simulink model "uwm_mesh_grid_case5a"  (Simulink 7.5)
settings: Solver=ode45  StartTime=0.0  StopTime=3.0  RelTol=1e-4
undefined symbols (not defined in the file or in its folder): D1, Delta, dfilt, DiscIntNeverNeededParam, Discrete, no, powergui, steady, ZData
libraries: powerlib x259, powerlib_extras x68, dsparch4 x11
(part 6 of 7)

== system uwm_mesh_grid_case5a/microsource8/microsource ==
  Vpk : Inport  OutDataType=fixdt(1, 16)  OutScaling=2^0
  w : Inport  Port=2  OutDataType=fixdt(1, 16)  OutScaling=2^0
  Demux : Demux  Outputs=3
  Ground2 : powerlib/Elements/Ground  DialogController=POWERSYS.PowerSysDialog  PhysicalDomain=powersysdomain  SubClassName=unknown  LeftPortType=p1  RightPortType=p1  LConnTagsString=a
  Integrator : Integrator
  Mux : Mux  Inputs=3
  Product : Product  OutDataType=sfix(16)  OutScaling=2^0
  Series RLC Branch : powerlib/Elements/Series RLC Branch  DialogController=POWERSYS.PowerSysDialog  PhysicalDomain=powersysdomain  SubClassName=unknown  LeftPortType=p1  RightPortType=p1  LConnTagsString=__new0  RConnTagsString=__new0  BranchType=C  Resistance=1  Inductance=1e-3  SetiL0=off  InitialCurrent=0  Capacitance=1e-8  Setx0=off  InitialVoltage=0  Measurements=None
  phaseA : powerlib/Electrical Sources/Controlled Voltage Source  DialogController=POWERSYS.PowerSysDialog  SystemSampleTime=-1  Initialize=on  Source_Type=AC  Amplitude=0  Phase=0  Frequency=0  Measurements=None
  phaseB : powerlib/Electrical Sources/Controlled Voltage Source  DialogController=POWERSYS.PowerSysDialog  SystemSampleTime=-1  Initialize=on  Source_Type=AC  Amplitude=0  Phase=0  Frequency=0  Measurements=None
  phaseC : powerlib/Electrical Sources/Controlled Voltage Source  DialogController=POWERSYS.PowerSysDialog  SystemSampleTime=-1  Initialize=on  Source_Type=AC  Amplitude=0  Phase=0  Frequency=0  Measurements=None
  v_A : Fcn  Expr=cos(u)
  v_B : Fcn  Expr=cos(u-2*pi/3)
  v_C : Fcn  Expr=cos(u+2*pi/3)
  Va : PMIOPort  Tag=PMCPort  Port=1  Side=Right
  Vb : PMIOPort  Tag=PMCPort  Port=2  Side=Right
  Vc : PMIOPort  Tag=PMCPort  Port=3  Side=Right
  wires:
  Product/1 -> Demux/1
  Vpk/1 -> Product/1
  Mux/1 -> Product/2
  w/1 -> Integrator/1
  Integrator/1 -> v_A/1, v_B/1, v_C/1
  v_A/1 -> Mux/1
  v_B/1 -> Mux/2
  v_C/1 -> Mux/3
  Demux/1 -> phaseA/1
  Demux/2 -> phaseB/1
  Demux/3 -> phaseC/1
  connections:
  Vb/RConn1 -- phaseB/RConn1 -- phaseA/LConn1
  Va/RConn1 -- phaseC/LConn1 -- phaseA/RConn1
  Vc/RConn1 -- phaseC/RConn1
  Series RLC Branch/RConn1 -- Ground2/LConn1
  Series RLC Branch/LConn1 -- phaseB/LConn1

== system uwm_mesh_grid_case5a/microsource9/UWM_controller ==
  note: P
  note: Q
  v_meas : Inport
  i_meas : Inport  Port=2
  E_req : Inport  Port=3
  P_req : Inport  Port=4
  " pu convert P" : Gain  Gain=1/Sbase  ParameterDataType=sfix(16)  ParameterScaling=2^0  OutDataType=sfix(16)  OutScaling=2^0
  " pu convert S" : Gain  Gain=1/Sbase  ParameterDataType=sfix(16)  ParameterScaling=2^0  OutDataType=sfix(16)  OutScaling=2^0
  " pu convert V" : Gain  Gain=1/(Vbase/sqrt(3))  ParameterDataType=sfix(16)  ParameterScaling=2^0  OutDataType=sfix(16)  OutScaling=2^0
  3-phase  Instantaneous  Active & Reactive Power : powerlib_extras/Measurements/3-phase  Instantaneous  Active & Reactive Power  DialogController=POWERSYS.PowerSysDialog  SystemSampleTime=-1
  Demux : Demux  Outputs=2
  PI-Control : Subsystem
  RMS : Fcn  Expr=sqrt(u(1)*u(1)+u(2)*u(2)+u(3)*u(3))/sqrt(3)
  Sum : Sum  Inputs=|-+  OutDataType=sfix(16)  OutScaling=2^0
  Sum1 : Sum  Inputs=|+-  OutDataType=sfix(16)  OutScaling=2^0
  Sum2 : Sum  Inputs=+-|  OutDataType=sfix(16)  OutScaling=2^0
  Sum3 : Sum  Inputs=+++  OutDataType=sfix(16)  OutScaling=2^0
  Transfer Fcn : TransferFcn  Denominator=[.01 1]
  Transfer Fcn1 : TransferFcn  Denominator=[.01 1]
  Transfer Fcn2 : TransferFcn  Denominator=[.01 1]
  k : Gain  Gain=1/pi  ParameterDataType=sfix(16)  ParameterScaling=2^0  OutDataType=sfix(16)  OutScaling=2^0
  limiter : Subsystem
  mP droop : Gain  Gain=pi  ParameterDataType=sfix(16)  ParameterScaling=2^0  OutDataType=sfix(16)  OutScaling=2^0
  "mQ droop " : Gain  Gain=0.05  ParameterDataType=sfix(16)  ParameterScaling=2^0  OutDataType=sfix(16)  OutScaling=2^0
  w0 : Constant  Value=60*2*pi  OutDataType=fixdt(1, 16)  OutScaling=2^0
  Vpk : Outport
  w : Outport  Port=2
  Pmm : Outport  Port=3
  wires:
  Transfer Fcn2/1 -> " pu convert V"/1
  Transfer Fcn/1 -> " pu convert P"/1
  " pu convert P"/1 -> "mQ droop "/1
  Transfer Fcn1/1 -> " pu convert S"/1
  " pu convert S"/1 -> limiter/1(In1), Sum2/2
  i_meas/1 -> 3-phase  Instantaneous  Active & Reactive Power/2
  P_req/1 -> Sum2/1
  mP droop/1 -> Sum3/2
  limiter/1(Out1) -> Sum3/1, k/1
  w0/1 -> Sum3/3
  Sum2/1 -> mP droop/1
  Sum1/1 -> PI-Control/1(In1)
  Sum/1 -> Sum1/1
  "mQ droop "/1 -> Sum/1
  RMS/1 -> Transfer Fcn2/1
  Demux/2 -> Transfer Fcn/1
  Demux/1 -> Transfer Fcn1/1
  3-phase  Instantaneous  Active & Reactive Power/1 -> Demux/1
  v_meas/1 -> RMS/1, 3-phase  Instantaneous  Active & Reactive Power/1
  PI-Control/1(Out1) -> Vpk/1
  Sum3/1 -> w/1
  E_req/1 -> Sum/2
  " pu convert V"/1 -> Sum1/2
  k/1 -> Pmm/1

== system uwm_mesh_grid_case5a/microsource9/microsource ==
  Vpk : Inport  OutDataType=fixdt(1, 16)  OutScaling=2^0
  w : Inport  Port=2  OutDataType=fixdt(1, 16)  OutScaling=2^0
  Demux : Demux  Outputs=3
  Ground2 : powerlib/Elements/Ground  DialogController=POWERSYS.PowerSysDialog  PhysicalDomain=powersysdomain  SubClassName=unknown  LeftPortType=p1  RightPortType=p1  LConnTagsString=a
  Integrator : Integrator
  Mux : Mux  Inputs=3
  Product : Product  OutDataType=sfix(16)  OutScaling=2^0
  Series RLC Branch : powerlib/Elements/Series RLC Branch  DialogController=POWERSYS.PowerSysDialog  PhysicalDomain=powersysdomain  SubClassName=unknown  LeftPortType=p1  RightPortType=p1  LConnTagsString=__new0  RConnTagsString=__new0  BranchType=C  Resistance=1  Inductance=1e-3  SetiL0=off  InitialCurrent=0  Capacitance=1e-8  Setx0=off  InitialVoltage=0  Measurements=None
  phaseA : powerlib/Electrical Sources/Controlled Voltage Source  DialogController=POWERSYS.PowerSysDialog  SystemSampleTime=-1  Initialize=on  Source_Type=AC  Amplitude=0  Phase=0  Frequency=0  Measurements=None
  phaseB : powerlib/Electrical Sources/Controlled Voltage Source  DialogController=POWERSYS.PowerSysDialog  SystemSampleTime=-1  Initialize=on  Source_Type=AC  Amplitude=0  Phase=0  Frequency=0  Measurements=None
  phaseC : powerlib/Electrical Sources/Controlled Voltage Source  DialogController=POWERSYS.PowerSysDialog  SystemSampleTime=-1  Initialize=on  Source_Type=AC  Amplitude=0  Phase=0  Frequency=0  Measurements=None
  v_A : Fcn  Expr=cos(u)
  v_B : Fcn  Expr=cos(u-2*pi/3)
  v_C : Fcn  Expr=cos(u+2*pi/3)
  Va : PMIOPort  Tag=PMCPort  Port=1  Side=Right
  Vb : PMIOPort  Tag=PMCPort  Port=2  Side=Right
  Vc : PMIOPort  Tag=PMCPort  Port=3  Side=Right
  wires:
  Product/1 -> Demux/1
  Vpk/1 -> Product/1
  Mux/1 -> Product/2
  w/1 -> Integrator/1
  Integrator/1 -> v_A/1, v_B/1, v_C/1
  v_A/1 -> Mux/1
  v_B/1 -> Mux/2
  v_C/1 -> Mux/3
  Demux/1 -> phaseA/1
  Demux/2 -> phaseB/1
  Demux/3 -> phaseC/1
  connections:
  Vb/RConn1 -- phaseB/RConn1 -- phaseA/LConn1
  Va/RConn1 -- phaseC/LConn1 -- phaseA/RConn1
  Vc/RConn1 -- phaseC/RConn1
  Series RLC Branch/RConn1 -- Ground2/LConn1
  Series RLC Branch/LConn1 -- phaseB/LConn1

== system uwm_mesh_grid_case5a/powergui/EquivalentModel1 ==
  Gates : Subsystem
  Sources : Subsystem
  State-Space : S-Function  FunctionName=sfun_spssw_discc  Parameters=S.Ts,S.A, S.B, S.C, S.D, S.x0, S.EnableUseOfTLC,S.SwitchResistance ,S.SwitchType, S.SwitchGateInitialValue, S.OutputsToResetToZero  EnableBusSupport=off
  Status : Subsystem
  Yout : Subsystem
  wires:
  State-Space/1 -> Yout/1(v,i)
  State-Space/2 -> Status/1(status)
  Sources/1(u) -> State-Space/1
  Gates/1(gates) -> State-Space/2

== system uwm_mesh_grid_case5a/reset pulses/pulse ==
  Step : Step  Time=tstart  SampleTime=0
  Step1 : Step  Time=tstart+dt  After=-1  SampleTime=0
  Sum : Sum  Inputs=|++  OutDataType=fixdt(1, 16)  OutScaling=2^0
  Out1 : Outport
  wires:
  Step/1 -> Sum/2
  Step1/1 -> Sum/1
  Sum/1 -> Out1/1

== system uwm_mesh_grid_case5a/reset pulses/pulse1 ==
  Step : Step  Time=tstart  SampleTime=0
  Step1 : Step  Time=tstart+dt  After=-1  SampleTime=0
  Sum : Sum  Inputs=|++  OutDataType=fixdt(1, 16)  OutScaling=2^0
  Out1 : Outport
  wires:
  Step/1 -> Sum/2
  Step1/1 -> Sum/1
  Sum/1 -> Out1/1

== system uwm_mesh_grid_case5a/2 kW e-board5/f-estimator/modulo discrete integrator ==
  In1 : Inport
  Abs : Abs
  Constant1 : Constant  OutDataType=sfix(16)  OutScaling=2^0
  Discrete-Time Integrator : DiscreteIntegrator  ExternalReset=rising  InitialConditionSource=external  SampleTime=dt  OutDataType=fixdt(1, 16)  OutScaling=2^0  UpperSaturationLimit=100  LowerSaturationLimit=-100  ShowStatePort=on  ICPrevOutput=DiscIntNeverNeededParam  ICPrevScaledInput=DiscIntNeverNeededParam
  Gain1 : Gain  Gain=1+.0001  ParameterDataType=sfix(16)  ParameterScaling=2^0  OutDataType=sfix(16)  OutScaling=2^0
  IC : InitialCondition  Value=0
  Math Function : Math  Operator=rem  OutDataType=sfix(16)  OutScaling=2^0
  Relational Operator : RelationalOperator
  Out1 : Outport
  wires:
  Math Function/1 -> IC/1
  IC/1 -> Discrete-Time Integrator/3
  Discrete-Time Integrator/1 -> Out1/1
  In1/1 -> Discrete-Time Integrator/1
  Abs/1 -> Math Function/1, Relational Operator/1
  Constant1/1 -> Math Function/2, Relational Operator/2
  Gain1/1 -> Abs/1
  Discrete-Time Integrator/State -> Gain1/1
  Relational Operator/1 -> Discrete-Time Integrator/2

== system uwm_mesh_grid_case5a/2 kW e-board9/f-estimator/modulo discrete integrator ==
  In1 : Inport
  Abs : Abs
  Constant1 : Constant  OutDataType=sfix(16)  OutScaling=2^0
  Discrete-Time Integrator : DiscreteIntegrator  ExternalReset=rising  InitialConditionSource=external  SampleTime=dt  OutDataType=fixdt(1, 16)  OutScaling=2^0  UpperSaturationLimit=100  LowerSaturationLimit=-100  ShowStatePort=on  ICPrevOutput=DiscIntNeverNeededParam  ICPrevScaledInput=DiscIntNeverNeededParam
  Gain1 : Gain  Gain=1+.0001  ParameterDataType=sfix(16)  ParameterScaling=2^0  OutDataType=sfix(16)  OutScaling=2^0
  IC : InitialCondition  Value=0
  Math Function : Math  Operator=rem  OutDataType=sfix(16)  OutScaling=2^0
  Relational Operator : RelationalOperator
  Out1 : Outport
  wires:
  Math Function/1 -> IC/1
  IC/1 -> Discrete-Time Integrator/3
  Discrete-Time Integrator/1 -> Out1/1
  In1/1 -> Discrete-Time Integrator/1
  Abs/1 -> Math Function/1, Relational Operator/1
  Constant1/1 -> Math Function/2, Relational Operator/2
  Gain1/1 -> Abs/1
  Discrete-Time Integrator/State -> Gain1/1
  Relational Operator/1 -> Discrete-Time Integrator/2

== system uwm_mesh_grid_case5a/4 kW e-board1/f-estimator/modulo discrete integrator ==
  In1 : Inport
  Abs : Abs
  Constant1 : Constant  OutDataType=sfix(16)  OutScaling=2^0
  Discrete-Time Integrator : DiscreteIntegrator  ExternalReset=rising  InitialConditionSource=external  SampleTime=dt  OutDataType=fixdt(1, 16)  OutScaling=2^0  UpperSaturationLimit=100  LowerSaturationLimit=-100  ShowStatePort=on  ICPrevOutput=DiscIntNeverNeededParam  ICPrevScaledInput=DiscIntNeverNeededParam
  Gain1 : Gain  Gain=1+.0001  ParameterDataType=sfix(16)  ParameterScaling=2^0  OutDataType=sfix(16)  OutScaling=2^0
  IC : InitialCondition  Value=0
  Math Function : Math  Operator=rem  OutDataType=sfix(16)  OutScaling=2^0
  Relational Operator : RelationalOperator
  Out1 : Outport
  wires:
  Math Function/1 -> IC/1
  IC/1 -> Discrete-Time Integrator/3
  Discrete-Time Integrator/1 -> Out1/1
  In1/1 -> Discrete-Time Integrator/1
  Abs/1 -> Math Function/1, Relational Operator/1
  Constant1/1 -> Math Function/2, Relational Operator/2
  Gain1/1 -> Abs/1
  Discrete-Time Integrator/State -> Gain1/1
  Relational Operator/1 -> Discrete-Time Integrator/2

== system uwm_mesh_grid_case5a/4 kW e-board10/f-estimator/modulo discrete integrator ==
  In1 : Inport
  Abs : Abs
  Constant1 : Constant  OutDataType=sfix(16)  OutScaling=2^0
  Discrete-Time Integrator : DiscreteIntegrator  ExternalReset=rising  InitialConditionSource=external  SampleTime=dt  OutDataType=fixdt(1, 16)  OutScaling=2^0  UpperSaturationLimit=100  LowerSaturationLimit=-100  ShowStatePort=on  ICPrevOutput=DiscIntNeverNeededParam  ICPrevScaledInput=DiscIntNeverNeededParam
  Gain1 : Gain  Gain=1+.0001  ParameterDataType=sfix(16)  ParameterScaling=2^0  OutDataType=sfix(16)  OutScaling=2^0
  IC : InitialCondition  Value=0
  Math Function : Math  Operator=rem  OutDataType=sfix(16)  OutScaling=2^0
  Relational Operator : RelationalOperator
  Out1 : Outport
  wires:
  Math Function/1 -> IC/1
  IC/1 -> Discrete-Time Integrator/3
  Discrete-Time Integrator/1 -> Out1/1
  In1/1 -> Discrete-Time Integrator/1
  Abs/1 -> Math Function/1, Relational Operator/1
  Constant1/1 -> Math Function/2, Relational Operator/2
  Gain1/1 -> Abs/1
  Discrete-Time Integrator/State -> Gain1/1
  Relational Operator/1 -> Discrete-Time Integrator/2

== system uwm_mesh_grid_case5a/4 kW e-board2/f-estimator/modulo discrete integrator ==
  In1 : Inport
  Abs : Abs
  Constant1 : Constant  OutDataType=sfix(16)  OutScaling=2^0
  Discrete-Time Integrator : DiscreteIntegrator  ExternalReset=rising  InitialConditionSource=external  SampleTime=dt  OutDataType=fixdt(1, 16)  OutScaling=2^0  UpperSaturationLimit=100  LowerSaturationLimit=-100  ShowStatePort=on  ICPrevOutput=DiscIntNeverNeededParam  ICPrevScaledInput=DiscIntNeverNeededParam
  Gain1 : Gain  Gain=1+.0001  ParameterDataType=sfix(16)  ParameterScaling=2^0  OutDataType=sfix(16)  OutScaling=2^0
  IC : InitialCondition  Value=0
  Math Function : Math  Operator=rem  OutDataType=sfix(16)  OutScaling=2^0
  Relational Operator : RelationalOperator
  Out1 : Outport
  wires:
  Math Function/1 -> IC/1
  IC/1 -> Discrete-Time Integrator/3
  Discrete-Time Integrator/1 -> Out1/1
  In1/1 -> Discrete-Time Integrator/1
  Abs/1 -> Math Function/1, Relational Operator/1
  Constant1/1 -> Math Function/2, Relational Operator/2
  Gain1/1 -> Abs/1
  Discrete-Time Integrator/State -> Gain1/1
  Relational Operator/1 -> Discrete-Time Integrator/2

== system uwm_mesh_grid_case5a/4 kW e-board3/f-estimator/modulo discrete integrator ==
  In1 : Inport
  Abs : Abs
  Constant1 : Constant  OutDataType=sfix(16)  OutScaling=2^0
  Discrete-Time Integrator : DiscreteIntegrator  ExternalReset=rising  InitialConditionSource=external  SampleTime=dt  OutDataType=fixdt(1, 16)  OutScaling=2^0  UpperSaturationLimit=100  LowerSaturationLimit=-100  ShowStatePort=on  ICPrevOutput=DiscIntNeverNeededParam  ICPrevScaledInput=DiscIntNeverNeededParam
  Gain1 : Gain  Gain=1+.0001  ParameterDataType=sfix(16)  ParameterScaling=2^0  OutDataType=sfix(16)  OutScaling=2^0
  IC : InitialCondition  Value=0
  Math Function : Math  Operator=rem  OutDataType=sfix(16)  OutScaling=2^0
  Relational Operator : RelationalOperator
  Out1 : Outport
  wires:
  Math Function/1 -> IC/1
  IC/1 -> Discrete-Time Integrator/3
  Discrete-Time Integrator/1 -> Out1/1
  In1/1 -> Discrete-Time Integrator/1
  Abs/1 -> Math Function/1, Relational Operator/1
  Constant1/1 -> Math Function/2, Relational Operator/2
  Gain1/1 -> Abs/1
  Discrete-Time Integrator/State -> Gain1/1
  Relational Operator/1 -> Discrete-Time Integrator/2

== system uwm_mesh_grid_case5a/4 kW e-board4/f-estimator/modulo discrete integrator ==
  In1 : Inport
  Abs : Abs
  Constant1 : Constant  OutDataType=sfix(16)  OutScaling=2^0
  Discrete-Time Integrator : DiscreteIntegrator  ExternalReset=rising  InitialConditionSource=external  SampleTime=dt  OutDataType=fixdt(1, 16)  OutScaling=2^0  UpperSaturationLimit=100  LowerSaturationLimit=-100  ShowStatePort=on  ICPrevOutput=DiscIntNeverNeededParam  ICPrevScaledInput=DiscIntNeverNeededParam
  Gain1 : Gain  Gain=1+.0001  ParameterDataType=sfix(16)  ParameterScaling=2^0  OutDataType=sfix(16)  OutScaling=2^0
  IC : InitialCondition  Value=0
  Math Function : Math  Operator=rem  OutDataType=sfix(16)  OutScaling=2^0
  Relational Operator : RelationalOperator
  Out1 : Outport
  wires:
  Math Function/1 -> IC/1
  IC/1 -> Discrete-Time Integrator/3
  Discrete-Time Integrator/1 -> Out1/1
  In1/1 -> Discrete-Time Integrator/1
  Abs/1 -> Math Function/1, Relational Operator/1
  Constant1/1 -> Math Function/2, Relational Operator/2
  Gain1/1 -> Abs/1
  Discrete-Time Integrator/State -> Gain1/1
  Relational Operator/1 -> Discrete-Time Integrator/2

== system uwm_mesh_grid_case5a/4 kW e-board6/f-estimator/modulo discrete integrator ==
  In1 : Inport
  Abs : Abs
  Constant1 : Constant  OutDataType=sfix(16)  OutScaling=2^0
  Discrete-Time Integrator : DiscreteIntegrator  ExternalReset=rising  InitialConditionSource=external  SampleTime=dt  OutDataType=fixdt(1, 16)  OutScaling=2^0  UpperSaturationLimit=100  LowerSaturationLimit=-100  ShowStatePort=on  ICPrevOutput=DiscIntNeverNeededParam  ICPrevScaledInput=DiscIntNeverNeededParam
  Gain1 : Gain  Gain=1+.0001  ParameterDataType=sfix(16)  ParameterScaling=2^0  OutDataType=sfix(16)  OutScaling=2^0
  IC : InitialCondition  Value=0
  Math Function : Math  Operator=rem  OutDataType=sfix(16)  OutScaling=2^0
  Relational Operator : RelationalOperator
  Out1 : Outport
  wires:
  Math Function/1 -> IC/1
  IC/1 -> Discrete-Time Integrator/3
  Discrete-Time Integrator/1 -> Out1/1
  In1/1 -> Discrete-Time Integrator/1
  Abs/1 -> Math Function/1, Relational Operator/1
  Constant1/1 -> Math Function/2, Relational Operator/2
  Gain1/1 -> Abs/1
  Discrete-Time Integrator/State -> Gain1/1
  Relational Operator/1 -> Discrete-Time Integrator/2

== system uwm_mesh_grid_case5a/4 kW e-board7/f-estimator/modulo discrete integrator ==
  In1 : Inport
  Abs : Abs
  Constant1 : Constant  OutDataType=sfix(16)  OutScaling=2^0
  Discrete-Time Integrator : DiscreteIntegrator  ExternalReset=rising  InitialConditionSource=external  SampleTime=dt  OutDataType=fixdt(1, 16)  OutScaling=2^0  UpperSaturationLimit=100  LowerSaturationLimit=-100  ShowStatePort=on  ICPrevOutput=DiscIntNeverNeededParam  ICPrevScaledInput=DiscIntNeverNeededParam
  Gain1 : Gain  Gain=1+.0001  ParameterDataType=sfix(16)  ParameterScaling=2^0  OutDataType=sfix(16)  OutScaling=2^0
  IC : InitialCondition  Value=0
  Math Function : Math  Operator=rem  OutDataType=sfix(16)  OutScaling=2^0
  Relational Operator : RelationalOperator
  Out1 : Outport
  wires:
  Math Function/1 -> IC/1
  IC/1 -> Discrete-Time Integrator/3
  Discrete-Time Integrator/1 -> Out1/1
  In1/1 -> Discrete-Time Integrator/1
  Abs/1 -> Math Function/1, Relational Operator/1
  Constant1/1 -> Math Function/2, Relational Operator/2
  Gain1/1 -> Abs/1
  Discrete-Time Integrator/State -> Gain1/1
  Relational Operator/1 -> Discrete-Time Integrator/2

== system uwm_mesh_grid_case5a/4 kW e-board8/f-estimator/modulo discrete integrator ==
  In1 : Inport
  Abs : Abs
  Constant1 : Constant  OutDataType=sfix(16)  OutScaling=2^0
  Discrete-Time Integrator : DiscreteIntegrator  ExternalReset=rising  InitialConditionSource=external  SampleTime=dt  OutDataType=fixdt(1, 16)  OutScaling=2^0  UpperSaturationLimit=100  LowerSaturationLimit=-100  ShowStatePort=on  ICPrevOutput=DiscIntNeverNeededParam  ICPrevScaledInput=DiscIntNeverNeededParam
  Gain1 : Gain  Gain=1+.0001  ParameterDataType=sfix(16)  ParameterScaling=2^0  OutDataType=sfix(16)  OutScaling=2^0
  IC : InitialCondition  Value=0
  Math Function : Math  Operator=rem  OutDataType=sfix(16)  OutScaling=2^0
  Relational Operator : RelationalOperator
  Out1 : Outport
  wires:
  Math Function/1 -> IC/1
  IC/1 -> Discrete-Time Integrator/3
  Discrete-Time Integrator/1 -> Out1/1
  In1/1 -> Discrete-Time Integrator/1
  Abs/1 -> Math Function/1, Relational Operator/1
  Constant1/1 -> Math Function/2, Relational Operator/2
  Gain1/1 -> Abs/1
  Discrete-Time Integrator/State -> Gain1/1
  Relational Operator/1 -> Discrete-Time Integrator/2

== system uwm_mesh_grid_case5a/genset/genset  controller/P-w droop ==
  note: P
  P_req : Inport
  P : Inport  Port=2
  Sum2 : Sum  Inputs=+-|  OutDataType=sfix(16)  OutScaling=2^0
  Sum3 : Sum  Inputs=+++  OutDataType=sfix(16)  OutScaling=2^0
  k : Gain  Gain=1/pi  ParameterDataType=sfix(16)  ParameterScaling=2^0  OutDataType=sfix(16)  OutScaling=2^0
  limiter : Subsystem
  mP droop : Gain  Gain=pi  ParameterDataType=sfix(16)  ParameterScaling=2^0  OutDataType=sfix(16)  OutScaling=2^0
  rad2pu : Gain  Gain=1/(2*pi*60)  ParameterDataType=sfix(16)  ParameterScaling=2^0  OutDataType=sfix(16)  OutScaling=2^0
  w0 : Constant  Value=60*2*pi  OutDataType=fixdt(1, 16)  OutScaling=2^0
  w : Outport
  Pmm : Outport  Port=2
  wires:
  P_req/1 -> Sum2/1
  mP droop/1 -> Sum3/2
  limiter/1(Out1) -> Sum3/1, k/1
  w0/1 -> Sum3/3
  Sum2/1 -> mP droop/1
  P/1 -> limiter/1(In1), Sum2/2
  Sum3/1 -> rad2pu/1
  rad2pu/1 -> w/1
  k/1 -> Pmm/1

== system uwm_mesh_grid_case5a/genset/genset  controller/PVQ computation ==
  note: P
  note: Q
  Vabc : Inport  OutDataType=fixdt(1, 16)  OutScaling=2^0
  Iabc : Inport  Port=2  OutDataType=fixdt(1, 16)  OutScaling=2^0
  " pu convert P" : Gain  Gain=1/Sbase  ParameterDataType=sfix(16)  ParameterScaling=2^0  OutDataType=sfix(16)  OutScaling=2^0
  " pu convert S" : Gain  Gain=1/Sbase  ParameterDataType=sfix(16)  ParameterScaling=2^0  OutDataType=sfix(16)  OutScaling=2^0
  " pu convert V" : Gain  Gain=1/(Vbase/sqrt(3))  ParameterDataType=sfix(16)  ParameterScaling=2^0  OutDataType=sfix(16)  OutScaling=2^0
  3-phase  Instantaneous  Active & Reactive Power : powerlib_extras/Measurements/3-phase  Instantaneous  Active & Reactive Power  DialogController=POWERSYS.PowerSysDialog  SystemSampleTime=-1
  Demux : Demux  Outputs=2
  RMS : Fcn  Expr=sqrt(u(1)*u(1)+u(2)*u(2)+u(3)*u(3))/sqrt(3)
  Transfer Fcn1 : TransferFcn  Denominator=[.01 1]
  Transfer Fcn2 : TransferFcn  Denominator=[.01 1]
  Transfer Fcn3 : TransferFcn  Denominator=[.01 1]
  P_pu : Outport  OutDataType=fixdt(1, 16)  OutScaling=2^0
  Vt : Outport  Port=2  OutDataType=fixdt(1, 16)  OutScaling=2^0
  Q_pu : Outport  Port=3  OutDataType=fixdt(1, 16)  OutScaling=2^0
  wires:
  Iabc/1 -> 3-phase  Instantaneous  Active & Reactive Power/2
  RMS/1 -> " pu convert V"/1
  Demux/2 -> " pu convert P"/1
  Demux/1 -> " pu convert S"/1
  3-phase  Instantaneous  Active & Reactive Power/1 -> Demux/1
  Vabc/1 -> RMS/1, 3-phase  Instantaneous  Active & Reactive Power/1
  Transfer Fcn1/1 -> P_pu/1
  " pu convert S"/1 -> Transfer Fcn1/1
  Transfer Fcn2/1 -> Q_pu/1
  " pu convert P"/1 -> Transfer Fcn2/1
  Transfer Fcn3/1 -> Vt/1
  " pu convert V"/1 -> Transfer Fcn3/1

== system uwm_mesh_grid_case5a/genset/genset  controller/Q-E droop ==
  note: Q
  v_meas : Inport
  Q : Inport  Port=2
  E_req : Inport  Port=3
  PI-Control : Subsystem
  Sum : Sum  Inputs=|-+  OutDataType=sfix(16)  OutScaling=2^0
  Sum1 : Sum  Inputs=|+-  OutDataType=sfix(16)  OutScaling=2^0
  "mQ droop " : Gain  Gain=0.05  ParameterDataType=sfix(16)  ParameterScaling=2^0  OutDataType=sfix(16)  OutScaling=2^0
  Vpk : Outport
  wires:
  Sum1/1 -> PI-Control/1(In1)
  Sum/1 -> Sum1/1
  "mQ droop "/1 -> Sum/1
  PI-Control/1(Out1) -> Vpk/1
  Q/1 -> "mQ droop "/1
  E_req/1 -> Sum/2
  v_meas/1 -> Sum1/2

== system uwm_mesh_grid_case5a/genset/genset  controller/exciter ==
  wr : Inport  OutDataType=fixdt(1, 16)  OutScaling=2^0
  Ef_mcd_wr : Inport  Port=2  OutDataType=fixdt(1, 16)  OutScaling=2^0
  Product : Product  OutDataType=fixdt(1, 16)  OutScaling=2^0
  Saturation : Saturate  UpperLimit=10  LowerLimit=-10  OutDataType=fixdt(1, 16)  OutScaling=2^0
  Transfer Fcn : TransferFcn  Denominator=[.001 1]
  Ef : Outport  OutDataType=fixdt(1, 16)  OutScaling=2^0
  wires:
  wr/1 -> Product/2
  Ef_mcd_wr/1 -> Product/1
  Product/1 -> Saturation/1
  Saturation/1 -> Transfer Fcn/1
  Transfer Fcn/1 -> Ef/1

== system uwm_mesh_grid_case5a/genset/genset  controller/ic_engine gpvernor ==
  wr : Inport  OutDataType=fixdt(1, 16)  OutScaling=2^0
  Pmeas : Inport  Port=2  OutDataType=fixdt(1, 16)  OutScaling=2^0
  w : Inport  Port=3  OutDataType=fixdt(1, 16)  OutScaling=2^0
  IC_engine : Subsystem
  governor : Subsystem
  Pmech : Outport  OutDataType=fixdt(1, 16)  OutScaling=2^0
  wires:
  governor/1(fuel_cmd) -> IC_engine/1(fuel_cmd)
  Pmeas/1 -> governor/1(Pmeas)
  IC_engine/1(Pmech) -> Pmech/1
  wr/1 -> governor/3(wr), IC_engine/2(wr)
  w/1 -> governor/2(w)

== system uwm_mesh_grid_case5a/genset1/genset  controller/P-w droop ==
  note: P
  P_req : Inport
  P : Inport  Port=2
  Sum2 : Sum  Inputs=+-|  OutDataType=sfix(16)  OutScaling=2^0
  Sum3 : Sum  Inputs=+++  OutDataType=sfix(16)  OutScaling=2^0
  k : Gain  Gain=1/pi  ParameterDataType=sfix(16)  ParameterScaling=2^0  OutDataType=sfix(16)  OutScaling=2^0
  limiter : Subsystem
  mP droop : Gain  Gain=pi  ParameterDataType=sfix(16)  ParameterScaling=2^0  OutDataType=sfix(16)  OutScaling=2^0
  rad2pu : Gain  Gain=1/(2*pi*60)  ParameterDataType=sfix(16)  ParameterScaling=2^0  OutDataType=sfix(16)  OutScaling=2^0
  w0 : Constant  Value=60*2*pi  OutDataType=fixdt(1, 16)  OutScaling=2^0
  w : Outport
  Pmm : Outport  Port=2
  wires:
  P_req/1 -> Sum2/1
  mP droop/1 -> Sum3/2
  limiter/1(Out1) -> Sum3/1, k/1
  w0/1 -> Sum3/3
  Sum2/1 -> mP droop/1
  P/1 -> limiter/1(In1), Sum2/2
  Sum3/1 -> rad2pu/1
  rad2pu/1 -> w/1
  k/1 -> Pmm/1

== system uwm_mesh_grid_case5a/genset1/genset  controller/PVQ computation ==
  note: P
  note: Q
  Vabc : Inport  OutDataType=fixdt(1, 16)  OutScaling=2^0
  Iabc : Inport  Port=2  OutDataType=fixdt(1, 16)  OutScaling=2^0
  " pu convert P" : Gain  Gain=1/Sbase  ParameterDataType=sfix(16)  ParameterScaling=2^0  OutDataType=sfix(16)  OutScaling=2^0
  " pu convert S" : Gain  Gain=1/Sbase  ParameterDataType=sfix(16)  ParameterScaling=2^0  OutDataType=sfix(16)  OutScaling=2^0
  " pu convert V" : Gain  Gain=1/(Vbase/sqrt(3))  ParameterDataType=sfix(16)  ParameterScaling=2^0  OutDataType=sfix(16)  OutScaling=2^0
  3-phase  Instantaneous  Active & Reactive Power : powerlib_extras/Measurements/3-phase  Instantaneous  Active & Reactive Power  DialogController=POWERSYS.PowerSysDialog  SystemSampleTime=-1
  Demux : Demux  Outputs=2
  RMS : Fcn  Expr=sqrt(u(1)*u(1)+u(2)*u(2)+u(3)*u(3))/sqrt(3)
  Transfer Fcn1 : TransferFcn  Denominator=[.01 1]
  Transfer Fcn2 : TransferFcn  Denominator=[.01 1]
  Transfer Fcn3 : TransferFcn  Denominator=[.01 1]
  P_pu : Outport  OutDataType=fixdt(1, 16)  OutScaling=2^0
  Vt : Outport  Port=2  OutDataType=fixdt(1, 16)  OutScaling=2^0
  Q_pu : Outport  Port=3  OutDataType=fixdt(1, 16)  OutScaling=2^0
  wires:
  Iabc/1 -> 3-phase  Instantaneous  Active & Reactive Power/2
  RMS/1 -> " pu convert V"/1
  Demux/2 -> " pu convert P"/1
  Demux/1 -> " pu convert S"/1
  3-phase  Instantaneous  Active & Reactive Power/1 -> Demux/1
  Vabc/1 -> RMS/1, 3-phase  Instantaneous  Active & Reactive Power/1
  Transfer Fcn1/1 -> P_pu/1
  " pu convert S"/1 -> Transfer Fcn1/1
  Transfer Fcn2/1 -> Q_pu/1
  " pu convert P"/1 -> Transfer Fcn2/1
  Transfer Fcn3/1 -> Vt/1
  " pu convert V"/1 -> Transfer Fcn3/1

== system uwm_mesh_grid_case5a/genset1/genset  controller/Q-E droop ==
  note: Q
  v_meas : Inport
  Q : Inport  Port=2
  E_req : Inport  Port=3
  PI-Control : Subsystem
  Sum : Sum  Inputs=|-+  OutDataType=sfix(16)  OutScaling=2^0
  Sum1 : Sum  Inputs=|+-  OutDataType=sfix(16)  OutScaling=2^0
  "mQ droop " : Gain  Gain=0.05  ParameterDataType=sfix(16)  ParameterScaling=2^0  OutDataType=sfix(16)  OutScaling=2^0
  Vpk : Outport
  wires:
  Sum1/1 -> PI-Control/1(In1)
  Sum/1 -> Sum1/1
  "mQ droop "/1 -> Sum/1
  PI-Control/1(Out1) -> Vpk/1
  Q/1 -> "mQ droop "/1
  E_req/1 -> Sum/2
  v_meas/1 -> Sum1/2

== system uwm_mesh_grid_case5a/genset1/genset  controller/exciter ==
  wr : Inport  OutDataType=fixdt(1, 16)  OutScaling=2^0
  Ef_mcd_wr : Inport  Port=2  OutDataType=fixdt(1, 16)  OutScaling=2^0
  Product : Product  OutDataType=fixdt(1, 16)  OutScaling=2^0
  Saturation : Saturate  UpperLimit=10  LowerLimit=-10  OutDataType=fixdt(1, 16)  OutScaling=2^0
  Transfer Fcn : TransferFcn  Denominator=[.001 1]
  Ef : Outport  OutDataType=fixdt(1, 16)  OutScaling=2^0
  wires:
  wr/1 -> Product/2
  Ef_mcd_wr/1 -> Product/1
  Product/1 -> Saturation/1
  Saturation/1 -> Transfer Fcn/1
  Transfer Fcn/1 -> Ef/1

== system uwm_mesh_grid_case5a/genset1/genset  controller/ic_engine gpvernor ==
  wr : Inport  OutDataType=fixdt(1, 16)  OutScaling=2^0
  Pmeas : Inport  Port=2  OutDataType=fixdt(1, 16)  OutScaling=2^0
  w : Inport  Port=3  OutDataType=fixdt(1, 16)  OutScaling=2^0
  IC_engine : Subsystem
  governor : Subsystem
  Pmech : Outport  OutDataType=fixdt(1, 16)  OutScaling=2^0
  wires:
  governor/1(fuel_cmd) -> IC_engine/1(fuel_cmd)
  Pmeas/1 -> governor/1(Pmeas)
  IC_engine/1(Pmech) -> Pmech/1
  wr/1 -> governor/3(wr), IC_engine/2(wr)
  w/1 -> governor/2(w)

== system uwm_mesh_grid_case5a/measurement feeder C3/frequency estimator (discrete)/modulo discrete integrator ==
  In1 : Inport
  Abs : Abs
  Constant1 : Constant  OutDataType=sfix(16)  OutScaling=2^0
  Discrete-Time Integrator : DiscreteIntegrator  ExternalReset=rising  InitialConditionSource=external  SampleTime=dt  OutDataType=fixdt(1, 16)  OutScaling=2^0  UpperSaturationLimit=100  LowerSaturationLimit=-100  ShowStatePort=on  ICPrevOutput=DiscIntNeverNeededParam  ICPrevScaledInput=DiscIntNeverNeededParam
  Gain1 : Gain  Gain=1+.0001  ParameterDataType=sfix(16)  ParameterScaling=2^0  OutDataType=sfix(16)  OutScaling=2^0
  IC : InitialCondition  Value=0
  Math Function : Math  Operator=rem  OutDataType=sfix(16)  OutScaling=2^0
  Relational Operator : RelationalOperator
  Out1 : Outport
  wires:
  Relational Operator/1 -> Discrete-Time Integrator/2
  Discrete-Time Integrator/State -> Gain1/1
  Gain1/1 -> Abs/1
  Constant1/1 -> Relational Operator/2, Math Function/2
  Abs/1 -> Relational Operator/1, Math Function/1
  In1/1 -> Discrete-Time Integrator/1
  Discrete-Time Integrator/1 -> Out1/1
  IC/1 -> Discrete-Time Integrator/3
  Math Function/1 -> IC/1

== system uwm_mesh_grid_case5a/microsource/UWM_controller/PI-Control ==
  In1 : Inport
  Gain : Gain  Gain=.01  ParameterDataType=sfix(16)  ParameterScaling=2^0  OutDataType=sfix(16)  OutScaling=2^0
  Gain1 : Gain  Gain=5  ParameterDataType=sfix(16)  ParameterScaling=2^0  OutDataType=sfix(16)  OutScaling=2^0
  Gain2 : Gain  Gain=750  ParameterDataType=sfix(16)  ParameterScaling=2^0  OutDataType=sfix(16)  OutScaling=2^0
  Integrator1 : Integrator  LimitOutput=on  UpperSaturationLimit=100  LowerSaturationLimit=-100  ZeroCross=off
  Sum4 : Sum  Inputs=|++  OutDataType=sfix(16)  OutScaling=2^0
  Out1 : Outport
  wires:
  Gain/1 -> Sum4/1
  Integrator1/1 -> Sum4/2
  In1/1 -> Gain1/1, Gain/1
  Gain1/1 -> Integrator1/1
  Sum4/1 -> Gain2/1
  Gain2/1 -> Out1/1

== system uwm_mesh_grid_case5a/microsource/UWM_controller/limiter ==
  In1 : Inport
  Integrator1 : Integrator  LimitOutput=on  UpperSaturationLimit=0  LowerSaturationLimit=-pi  ZeroCross=off
  Integrator2 : Integrator  LimitOutput=on  UpperSaturationLimit=pi  LowerSaturationLimit=0  ZeroCross=off
  Kilim : Gain  Gain=30  ParameterDataType=sfix(16)  ParameterScaling=2^0  OutDataType=sfix(16)  OutScaling=2^0
  Kilim1 : Gain  Gain=30  ParameterDataType=sfix(16)  ParameterScaling=2^0  OutDataType=sfix(16)  OutScaling=2^0
  Kplim : Gain  Gain=3  ParameterDataType=sfix(16)  ParameterScaling=2^0  OutDataType=sfix(16)  OutScaling=2^0
  Kplim1 : Gain  Gain=3  ParameterDataType=sfix(16)  ParameterScaling=2^0  OutDataType=sfix(16)  OutScaling=2^0
  Plimit : Constant  Value=1.0  OutDataType=sfix(16)  OutScaling=2^0
  Plimit1 : Constant  Value=0.0  OutDataType=sfix(16)  OutScaling=2^0
  Saturation1 : Saturate  UpperLimit=pi  LowerLimit=0  OutDataType=fixdt(1, 16)  OutScaling=2^0
  Saturation2 : Saturate  UpperLimit=0  LowerLimit=-pi  OutDataType=fixdt(1, 16)  OutScaling=2^0
  Sum1 : Sum  Inputs=-+|  OutDataType=sfix(16)  OutScaling=2^0
  Sum2 : Sum  Inputs=|++  OutDataType=sfix(16)  OutScaling=2^0
  Sum3 : Sum  OutDataType=sfix(16)  OutScaling=2^0
  Sum4 : Sum  Inputs=|+-  OutDataType=sfix(16)  OutScaling=2^0
  Sum9 : Sum  Inputs=|++  OutDataType=sfix(16)  OutScaling=2^0
  Out1 : Outport
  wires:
  Sum3/1 -> Out1/1
  Plimit1/1 -> Sum1/2
  Integrator2/1 -> Sum2/2
  Kilim1/1 -> Integrator2/1
  Sum1/1 -> Kilim1/1, Kplim1/1
  In1/1 -> Sum1/1, Sum4/2
  Integrator1/1 -> Sum9/2
  Kilim/1 -> Integrator1/1
  Sum4/1 -> Kilim/1, Kplim/1
  Plimit/1 -> Sum4/1
  Kplim1/1 -> Saturation1/1
  Saturation1/1 -> Sum2/1
  Kplim/1 -> Saturation2/1
  Saturation2/1 -> Sum9/1
  Sum9/1 -> Sum3/1
  Sum2/1 -> Sum3/2

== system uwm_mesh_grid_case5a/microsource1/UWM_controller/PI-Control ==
  In1 : Inport
  Gain : Gain  Gain=.01  ParameterDataType=sfix(16)  ParameterScaling=2^0  OutDataType=sfix(16)  OutScaling=2^0
  Gain1 : Gain  Gain=5  ParameterDataType=sfix(16)  ParameterScaling=2^0  OutDataType=sfix(16)  OutScaling=2^0
  Gain2 : Gain  Gain=750  ParameterDataType=sfix(16)  ParameterScaling=2^0  OutDataType=sfix(16)  OutScaling=2^0
  Integrator1 : Integrator  LimitOutput=on  UpperSaturationLimit=100  LowerSaturationLimit=-100  ZeroCross=off
  Sum4 : Sum  Inputs=|++  OutDataType=sfix(16)  OutScaling=2^0
  Out1 : Outport
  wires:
  Gain/1 -> Sum4/1
  Integrator1/1 -> Sum4/2
  In1/1 -> Gain1/1, Gain/1
  Gain1/1 -> Integrator1/1
  Sum4/1 -> Gain2/1
  Gain2/1 -> Out1/1

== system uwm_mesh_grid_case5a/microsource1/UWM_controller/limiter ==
  In1 : Inport
  Integrator1 : Integrator  LimitOutput=on  UpperSaturationLimit=0  LowerSaturationLimit=-pi  ZeroCross=off
  Integrator2 : Integrator  LimitOutput=on  UpperSaturationLimit=pi  LowerSaturationLimit=0  ZeroCross=off
  Kilim : Gain  Gain=30  ParameterDataType=sfix(16)  ParameterScaling=2^0  OutDataType=sfix(16)  OutScaling=2^0
  Kilim1 : Gain  Gain=30  ParameterDataType=sfix(16)  ParameterScaling=2^0  OutDataType=sfix(16)  OutScaling=2^0
  Kplim : Gain  Gain=3  ParameterDataType=sfix(16)  ParameterScaling=2^0  OutDataType=sfix(16)  OutScaling=2^0
  Kplim1 : Gain  Gain=3  ParameterDataType=sfix(16)  ParameterScaling=2^0  OutDataType=sfix(16)  OutScaling=2^0
  Plimit : Constant  Value=1.0  OutDataType=sfix(16)  OutScaling=2^0
  Plimit1 : Constant  Value=0.0  OutDataType=sfix(16)  OutScaling=2^0
  Saturation1 : Saturate  UpperLimit=pi  LowerLimit=0  OutDataType=fixdt(1, 16)  OutScaling=2^0
  Saturation2 : Saturate  UpperLimit=0  LowerLimit=-pi  OutDataType=fixdt(1, 16)  OutScaling=2^0
  Sum1 : Sum  Inputs=-+|  OutDataType=sfix(16)  OutScaling=2^0
  Sum2 : Sum  Inputs=|++  OutDataType=sfix(16)  OutScaling=2^0
  Sum3 : Sum  OutDataType=sfix(16)  OutScaling=2^0
  Sum4 : Sum  Inputs=|+-  OutDataType=sfix(16)  OutScaling=2^0
  Sum9 : Sum  Inputs=|++  OutDataType=sfix(16)  OutScaling=2^0
  Out1 : Outport
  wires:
  Sum3/1 -> Out1/1
  Plimit1/1 -> Sum1/2
  Integrator2/1 -> Sum2/2
  Kilim1/1 -> Integrator2/1
  Sum1/1 -> Kilim1/1, Kplim1/1
  In1/1 -> Sum1/1, Sum4/2
  Integrator1/1 -> Sum9/2
  Kilim/1 -> Integrator1/1
  Sum4/1 -> Kilim/1, Kplim/1
  Plimit/1 -> Sum4/1
  Kplim1/1 -> Saturation1/1
  Saturation1/1 -> Sum2/1
  Kplim/1 -> Saturation2/1
  Saturation2/1 -> Sum9/1
  Sum9/1 -> Sum3/1
  Sum2/1 -> Sum3/2

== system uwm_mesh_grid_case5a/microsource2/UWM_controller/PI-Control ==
  In1 : Inport
  Gain : Gain  Gain=.01  ParameterDataType=sfix(16)  ParameterScaling=2^0  OutDataType=sfix(16)  OutScaling=2^0
  Gain1 : Gain  Gain=5  ParameterDataType=sfix(16)  ParameterScaling=2^0  OutDataType=sfix(16)  OutScaling=2^0
  Gain2 : Gain  Gain=750  ParameterDataType=sfix(16)  ParameterScaling=2^0  OutDataType=sfix(16)  OutScaling=2^0
  Integrator1 : Integrator  LimitOutput=on  UpperSaturationLimit=100  LowerSaturationLimit=-100  ZeroCross=off
  Sum4 : Sum  Inputs=|++  OutDataType=sfix(16)  OutScaling=2^0
  Out1 : Outport
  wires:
  Gain/1 -> Sum4/1
  Integrator1/1 -> Sum4/2
  In1/1 -> Gain1/1, Gain/1
  Gain1/1 -> Integrator1/1
  Sum4/1 -> Gain2/1
  Gain2/1 -> Out1/1

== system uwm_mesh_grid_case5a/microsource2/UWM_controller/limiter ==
  In1 : Inport
  Integrator1 : Integrator  LimitOutput=on  UpperSaturationLimit=0  LowerSaturationLimit=-pi  ZeroCross=off
  Integrator2 : Integrator  LimitOutput=on  UpperSaturationLimit=pi  LowerSaturationLimit=0  ZeroCross=off
  Kilim : Gain  Gain=30  ParameterDataType=sfix(16)  ParameterScaling=2^0  OutDataType=sfix(16)  OutScaling=2^0
  Kilim1 : Gain  Gain=30  ParameterDataType=sfix(16)  ParameterScaling=2^0  OutDataType=sfix(16)  OutScaling=2^0
  Kplim : Gain  Gain=3  ParameterDataType=sfix(16)  ParameterScaling=2^0  OutDataType=sfix(16)  OutScaling=2^0
  Kplim1 : Gain  Gain=3  ParameterDataType=sfix(16)  ParameterScaling=2^0  OutDataType=sfix(16)  OutScaling=2^0
  Plimit : Constant  Value=1.0  OutDataType=sfix(16)  OutScaling=2^0
  Plimit1 : Constant  Value=0.0  OutDataType=sfix(16)  OutScaling=2^0
  Saturation1 : Saturate  UpperLimit=pi  LowerLimit=0  OutDataType=fixdt(1, 16)  OutScaling=2^0
  Saturation2 : Saturate  UpperLimit=0  LowerLimit=-pi  OutDataType=fixdt(1, 16)  OutScaling=2^0
  Sum1 : Sum  Inputs=-+|  OutDataType=sfix(16)  OutScaling=2^0
  Sum2 : Sum  Inputs=|++  OutDataType=sfix(16)  OutScaling=2^0
  Sum3 : Sum  OutDataType=sfix(16)  OutScaling=2^0
  Sum4 : Sum  Inputs=|+-  OutDataType=sfix(16)  OutScaling=2^0
  Sum9 : Sum  Inputs=|++  OutDataType=sfix(16)  OutScaling=2^0
  Out1 : Outport
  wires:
  Sum3/1 -> Out1/1
  Plimit1/1 -> Sum1/2
  Integrator2/1 -> Sum2/2
  Kilim1/1 -> Integrator2/1
  Sum1/1 -> Kilim1/1, Kplim1/1
  In1/1 -> Sum1/1, Sum4/2
  Integrator1/1 -> Sum9/2
  Kilim/1 -> Integrator1/1
  Sum4/1 -> Kilim/1, Kplim/1
  Plimit/1 -> Sum4/1
  Kplim1/1 -> Saturation1/1
  Saturation1/1 -> Sum2/1
  Kplim/1 -> Saturation2/1
  Saturation2/1 -> Sum9/1
  Sum9/1 -> Sum3/1
  Sum2/1 -> Sum3/2

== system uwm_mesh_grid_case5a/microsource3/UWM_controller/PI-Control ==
  In1 : Inport
  Gain : Gain  Gain=.01  ParameterDataType=sfix(16)  ParameterScaling=2^0  OutDataType=sfix(16)  OutScaling=2^0
  Gain1 : Gain  Gain=5  ParameterDataType=sfix(16)  ParameterScaling=2^0  OutDataType=sfix(16)  OutScaling=2^0
  Gain2 : Gain  Gain=750  ParameterDataType=sfix(16)  ParameterScaling=2^0  OutDataType=sfix(16)  OutScaling=2^0
  Integrator1 : Integrator  LimitOutput=on  UpperSaturationLimit=100  LowerSaturationLimit=-100  ZeroCross=off
  Sum4 : Sum  Inputs=|++  OutDataType=sfix(16)  OutScaling=2^0
  Out1 : Outport
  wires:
  Gain/1 -> Sum4/1
  Integrator1/1 -> Sum4/2
  In1/1 -> Gain1/1, Gain/1
  Gain1/1 -> Integrator1/1
  Sum4/1 -> Gain2/1
  Gain2/1 -> Out1/1

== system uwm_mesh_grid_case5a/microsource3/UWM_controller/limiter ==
  In1 : Inport
  Integrator1 : Integrator  LimitOutput=on  UpperSaturationLimit=0  LowerSaturationLimit=-pi  ZeroCross=off
  Integrator2 : Integrator  LimitOutput=on  UpperSaturationLimit=pi  LowerSaturationLimit=0  ZeroCross=off
  Kilim : Gain  Gain=30  ParameterDataType=sfix(16)  ParameterScaling=2^0  OutDataType=sfix(16)  OutScaling=2^0
  Kilim1 : Gain  Gain=30  ParameterDataType=sfix(16)  ParameterScaling=2^0  OutDataType=sfix(16)  OutScaling=2^0
  Kplim : Gain  Gain=3  ParameterDataType=sfix(16)  ParameterScaling=2^0  OutDataType=sfix(16)  OutScaling=2^0
  Kplim1 : Gain  Gain=3  ParameterDataType=sfix(16)  ParameterScaling=2^0  OutDataType=sfix(16)  OutScaling=2^0
  Plimit : Constant  Value=1.0  OutDataType=sfix(16)  OutScaling=2^0
  Plimit1 : Constant  Value=0.0  OutDataType=sfix(16)  OutScaling=2^0
  Saturation1 : Saturate  UpperLimit=pi  LowerLimit=0  OutDataType=fixdt(1, 16)  OutScaling=2^0
  Saturation2 : Saturate  UpperLimit=0  LowerLimit=-pi  OutDataType=fixdt(1, 16)  OutScaling=2^0
  Sum1 : Sum  Inputs=-+|  OutDataType=sfix(16)  OutScaling=2^0
  Sum2 : Sum  Inputs=|++  OutDataType=sfix(16)  OutScaling=2^0
  Sum3 : Sum  OutDataType=sfix(16)  OutScaling=2^0
  Sum4 : Sum  Inputs=|+-  OutDataType=sfix(16)  OutScaling=2^0
  Sum9 : Sum  Inputs=|++  OutDataType=sfix(16)  OutScaling=2^0
  Out1 : Outport
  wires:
  Sum3/1 -> Out1/1
  Plimit1/1 -> Sum1/2
  Integrator2/1 -> Sum2/2
  Kilim1/1 -> Integrator2/1
  Sum1/1 -> Kilim1/1, Kplim1/1
  In1/1 -> Sum1/1, Sum4/2
  Integrator1/1 -> Sum9/2
  Kilim/1 -> Integrator1/1
  Sum4/1 -> Kilim/1, Kplim/1
  Plimit/1 -> Sum4/1
  Kplim1/1 -> Saturation1/1
  Saturation1/1 -> Sum2/1
  Kplim/1 -> Saturation2/1
  Saturation2/1 -> Sum9/1
  Sum9/1 -> Sum3/1
  Sum2/1 -> Sum3/2

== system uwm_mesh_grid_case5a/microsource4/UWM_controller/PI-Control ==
  In1 : Inport
  Gain : Gain  Gain=.01  ParameterDataType=sfix(16)  ParameterScaling=2^0  OutDataType=sfix(16)  OutScaling=2^0
  Gain1 : Gain  Gain=5  ParameterDataType=sfix(16)  ParameterScaling=2^0  OutDataType=sfix(16)  OutScaling=2^0
  Gain2 : Gain  Gain=750  ParameterDataType=sfix(16)  ParameterScaling=2^0  OutDataType=sfix(16)  OutScaling=2^0
  Integrator1 : Integrator  LimitOutput=on  UpperSaturationLimit=100  LowerSaturationLimit=-100  ZeroCross=off
  Sum4 : Sum  Inputs=|++  OutDataType=sfix(16)  OutScaling=2^0
  Out1 : Outport
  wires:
  Gain/1 -> Sum4/1
  Integrator1/1 -> Sum4/2
  In1/1 -> Gain1/1, Gain/1
  Gain1/1 -> Integrator1/1
  Sum4/1 -> Gain2/1
  Gain2/1 -> Out1/1

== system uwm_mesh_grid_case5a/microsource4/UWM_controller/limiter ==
  In1 : Inport
  Integrator1 : Integrator  LimitOutput=on  UpperSaturationLimit=0  LowerSaturationLimit=-pi  ZeroCross=off
  Integrator2 : Integrator  LimitOutput=on  UpperSaturationLimit=pi  LowerSaturationLimit=0  ZeroCross=off
  Kilim : Gain  Gain=30  ParameterDataType=sfix(16)  ParameterScaling=2^0  OutDataType=sfix(16)  OutScaling=2^0
  Kilim1 : Gain  Gain=30  ParameterDataType=sfix(16)  ParameterScaling=2^0  OutDataType=sfix(16)  OutScaling=2^0
  Kplim : Gain  Gain=3  ParameterDataType=sfix(16)  ParameterScaling=2^0  OutDataType=sfix(16)  OutScaling=2^0
  Kplim1 : Gain  Gain=3  ParameterDataType=sfix(16)  ParameterScaling=2^0  OutDataType=sfix(16)  OutScaling=2^0
  Plimit : Constant  Value=1.0  OutDataType=sfix(16)  OutScaling=2^0
  Plimit1 : Constant  Value=0.0  OutDataType=sfix(16)  OutScaling=2^0
  Saturation1 : Saturate  UpperLimit=pi  LowerLimit=0  OutDataType=fixdt(1, 16)  OutScaling=2^0
  Saturation2 : Saturate  UpperLimit=0  LowerLimit=-pi  OutDataType=fixdt(1, 16)  OutScaling=2^0
  Sum1 : Sum  Inputs=-+|  OutDataType=sfix(16)  OutScaling=2^0
  Sum2 : Sum  Inputs=|++  OutDataType=sfix(16)  OutScaling=2^0
  Sum3 : Sum  OutDataType=sfix(16)  OutScaling=2^0
  Sum4 : Sum  Inputs=|+-  OutDataType=sfix(16)  OutScaling=2^0
  Sum9 : Sum  Inputs=|++  OutDataType=sfix(16)  OutScaling=2^0
  Out1 : Outport
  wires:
  Sum3/1 -> Out1/1
  Plimit1/1 -> Sum1/2
  Integrator2/1 -> Sum2/2
  Kilim1/1 -> Integrator2/1
  Sum1/1 -> Kilim1/1, Kplim1/1
  In1/1 -> Sum1/1, Sum4/2
  Integrator1/1 -> Sum9/2
  Kilim/1 -> Integrator1/1
  Sum4/1 -> Kilim/1, Kplim/1
  Plimit/1 -> Sum4/1
  Kplim1/1 -> Saturation1/1
  Saturation1/1 -> Sum2/1
  Kplim/1 -> Saturation2/1
  Saturation2/1 -> Sum9/1
  Sum9/1 -> Sum3/1
  Sum2/1 -> Sum3/2

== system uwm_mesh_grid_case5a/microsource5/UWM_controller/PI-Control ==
  In1 : Inport
  Gain : Gain  Gain=.01  ParameterDataType=sfix(16)  ParameterScaling=2^0  OutDataType=sfix(16)  OutScaling=2^0
  Gain1 : Gain  Gain=5  ParameterDataType=sfix(16)  ParameterScaling=2^0  OutDataType=sfix(16)  OutScaling=2^0
  Gain2 : Gain  Gain=750  ParameterDataType=sfix(16)  ParameterScaling=2^0  OutDataType=sfix(16)  OutScaling=2^0
  Integrator1 : Integrator  LimitOutput=on  UpperSaturationLimit=100  LowerSaturationLimit=-100  ZeroCross=off
  Sum4 : Sum  Inputs=|++  OutDataType=sfix(16)  OutScaling=2^0
  Out1 : Outport
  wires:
  Gain/1 -> Sum4/1
  Integrator1/1 -> Sum4/2
  In1/1 -> Gain1/1, Gain/1
  Gain1/1 -> Integrator1/1
  Sum4/1 -> Gain2/1
  Gain2/1 -> Out1/1

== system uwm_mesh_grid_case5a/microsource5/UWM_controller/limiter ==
  In1 : Inport
  Integrator1 : Integrator  LimitOutput=on  UpperSaturationLimit=0  LowerSaturationLimit=-pi  ZeroCross=off
  Integrator2 : Integrator  LimitOutput=on  UpperSaturationLimit=pi  LowerSaturationLimit=0  ZeroCross=off
  Kilim : Gain  Gain=30  ParameterDataType=sfix(16)  ParameterScaling=2^0  OutDataType=sfix(16)  OutScaling=2^0
  Kilim1 : Gain  Gain=30  ParameterDataType=sfix(16)  ParameterScaling=2^0  OutDataType=sfix(16)  OutScaling=2^0
  Kplim : Gain  Gain=3  ParameterDataType=sfix(16)  ParameterScaling=2^0  OutDataType=sfix(16)  OutScaling=2^0
  Kplim1 : Gain  Gain=3  ParameterDataType=sfix(16)  ParameterScaling=2^0  OutDataType=sfix(16)  OutScaling=2^0
  Plimit : Constant  Value=1.0  OutDataType=sfix(16)  OutScaling=2^0
  Plimit1 : Constant  Value=0.0  OutDataType=sfix(16)  OutScaling=2^0
  Saturation1 : Saturate  UpperLimit=pi  LowerLimit=0  OutDataType=fixdt(1, 16)  OutScaling=2^0
  Saturation2 : Saturate  UpperLimit=0  LowerLimit=-pi  OutDataType=fixdt(1, 16)  OutScaling=2^0
  Sum1 : Sum  Inputs=-+|  OutDataType=sfix(16)  OutScaling=2^0
  Sum2 : Sum  Inputs=|++  OutDataType=sfix(16)  OutScaling=2^0
  Sum3 : Sum  OutDataType=sfix(16)  OutScaling=2^0
  Sum4 : Sum  Inputs=|+-  OutDataType=sfix(16)  OutScaling=2^0
  Sum9 : Sum  Inputs=|++  OutDataType=sfix(16)  OutScaling=2^0
  Out1 : Outport
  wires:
  Sum3/1 -> Out1/1
  Plimit1/1 -> Sum1/2
  Integrator2/1 -> Sum2/2
  Kilim1/1 -> Integrator2/1
  Sum1/1 -> Kilim1/1, Kplim1/1
  In1/1 -> Sum1/1, Sum4/2
  Integrator1/1 -> Sum9/2
  Kilim/1 -> Integrator1/1
  Sum4/1 -> Kilim/1, Kplim/1
  Plimit/1 -> Sum4/1
  Kplim1/1 -> Saturation1/1
  Saturation1/1 -> Sum2/1
  Kplim/1 -> Saturation2/1
  Saturation2/1 -> Sum9/1
  Sum9/1 -> Sum3/1
  Sum2/1 -> Sum3/2

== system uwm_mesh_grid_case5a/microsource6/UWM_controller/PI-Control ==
  In1 : Inport
  Gain : Gain  Gain=.01  ParameterDataType=sfix(16)  ParameterScaling=2^0  OutDataType=sfix(16)  OutScaling=2^0
  Gain1 : Gain  Gain=5  ParameterDataType=sfix(16)  ParameterScaling=2^0  OutDataType=sfix(16)  OutScaling=2^0
  Gain2 : Gain  Gain=750  ParameterDataType=sfix(16)  ParameterScaling=2^0  OutDataType=sfix(16)  OutScaling=2^0
  Integrator1 : Integrator  LimitOutput=on  UpperSaturationLimit=100  LowerSaturationLimit=-100  ZeroCross=off
  Sum4 : Sum  Inputs=|++  OutDataType=sfix(16)  OutScaling=2^0
  Out1 : Outport
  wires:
  Gain/1 -> Sum4/1
  Integrator1/1 -> Sum4/2
  In1/1 -> Gain1/1, Gain/1
  Gain1/1 -> Integrator1/1
  Sum4/1 -> Gain2/1
  Gain2/1 -> Out1/1

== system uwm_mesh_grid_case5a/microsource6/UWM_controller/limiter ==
  In1 : Inport
  Integrator1 : Integrator  LimitOutput=on  UpperSaturationLimit=0  LowerSaturationLimit=-pi  ZeroCross=off
  Integrator2 : Integrator  LimitOutput=on  UpperSaturationLimit=pi  LowerSaturationLimit=0  ZeroCross=off
  Kilim : Gain  Gain=30  ParameterDataType=sfix(16)  ParameterScaling=2^0  OutDataType=sfix(16)  OutScaling=2^0
  Kilim1 : Gain  Gain=30  ParameterDataType=sfix(16)  ParameterScaling=2^0  OutDataType=sfix(16)  OutScaling=2^0
  Kplim : Gain  Gain=3  ParameterDataType=sfix(16)  ParameterScaling=2^0  OutDataType=sfix(16)  OutScaling=2^0
  Kplim1 : Gain  Gain=3  ParameterDataType=sfix(16)  ParameterScaling=2^0  OutDataType=sfix(16)  OutScaling=2^0
  Plimit : Constant  Value=1.0  OutDataType=sfix(16)  OutScaling=2^0
  Plimit1 : Constant  Value=0.0  OutDataType=sfix(16)  OutScaling=2^0
  Saturation1 : Saturate  UpperLimit=pi  LowerLimit=0  OutDataType=fixdt(1, 16)  OutScaling=2^0
  Saturation2 : Saturate  UpperLimit=0  LowerLimit=-pi  OutDataType=fixdt(1, 16)  OutScaling=2^0
  Sum1 : Sum  Inputs=-+|  OutDataType=sfix(16)  OutScaling=2^0
  Sum2 : Sum  Inputs=|++  OutDataType=sfix(16)  OutScaling=2^0
  Sum3 : Sum  OutDataType=sfix(16)  OutScaling=2^0
  Sum4 : Sum  Inputs=|+-  OutDataType=sfix(16)  OutScaling=2^0
  Sum9 : Sum  Inputs=|++  OutDataType=sfix(16)  OutScaling=2^0
  Out1 : Outport
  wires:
  Sum3/1 -> Out1/1
  Plimit1/1 -> Sum1/2
  Integrator2/1 -> Sum2/2
  Kilim1/1 -> Integrator2/1
  Sum1/1 -> Kilim1/1, Kplim1/1
  In1/1 -> Sum1/1, Sum4/2
  Integrator1/1 -> Sum9/2
  Kilim/1 -> Integrator1/1
  Sum4/1 -> Kilim/1, Kplim/1
  Plimit/1 -> Sum4/1
  Kplim1/1 -> Saturation1/1
  Saturation1/1 -> Sum2/1
  Kplim/1 -> Saturation2/1
  Saturation2/1 -> Sum9/1
  Sum9/1 -> Sum3/1
  Sum2/1 -> Sum3/2

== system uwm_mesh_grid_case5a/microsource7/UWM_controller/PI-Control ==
  In1 : Inport
  Gain : Gain  Gain=.01  ParameterDataType=sfix(16)  ParameterScaling=2^0  OutDataType=sfix(16)  OutScaling=2^0
  Gain1 : Gain  Gain=5  ParameterDataType=sfix(16)  ParameterScaling=2^0  OutDataType=sfix(16)  OutScaling=2^0
  Gain2 : Gain  Gain=750  ParameterDataType=sfix(16)  ParameterScaling=2^0  OutDataType=sfix(16)  OutScaling=2^0
  Integrator1 : Integrator  LimitOutput=on  UpperSaturationLimit=100  LowerSaturationLimit=-100  ZeroCross=off
  Sum4 : Sum  Inputs=|++  OutDataType=sfix(16)  OutScaling=2^0
  Out1 : Outport
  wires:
  Gain/1 -> Sum4/1
  Integrator1/1 -> Sum4/2
  In1/1 -> Gain1/1, Gain/1
  Gain1/1 -> Integrator1/1
  Sum4/1 -> Gain2/1
  Gain2/1 -> Out1/1
